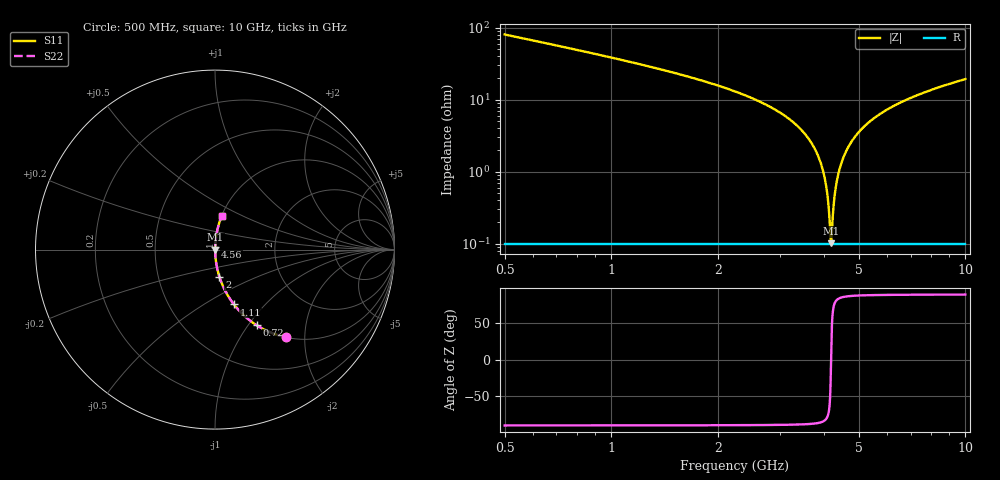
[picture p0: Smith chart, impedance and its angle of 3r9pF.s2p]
! Created Fri Jan 10 15:54:33 2014
# hz S db R 50
! 2 Port Network Data from SP1.SP block
! freq  dbS11  angS11  dbS21  angS21  dbS12  angS12  dbS22  angS22
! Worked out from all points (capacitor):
!   951 points, 500 MHz to 10 GHz, reference 50 ohm
!   read as one part in series: C = 3.9 pF near 540 MHz
!   lowest |Z| = 101 mohm at 4.18 GHz (marker M1)
!   series resonance near 4.176 GHz, so ESL is about 370 pH
!   S11 on the Smith chart (normalised r, x): 500 MHz: 1.00, -1.61; 720 MHz: 1.00, -1.10; 1.11 GHz: 1.00, -0.68; 2 GHz: 1.00, -0.31; 4.56 GHz: 1.00, +0.03; 10 GHz: 1.00, +0.39
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5e8  -4.06 -51.1  -2.17 38.8  -2.17 38.8  -4.06 -51.1
7.2e8  -6.35 -61.1  -1.15 28.8  -1.15 28.8  -6.35 -61.1
1.11e9  -9.82 -71.0  -0.49 18.8  -0.49 18.8  -9.82 -71.0
2e9  -16.18 -80.7  -0.11 8.9  -0.11 8.9  -16.18 -80.7
2.09e9  -16.79 -81.3  -0.10 8.3  -0.10 8.3  -16.79 -81.3
3.09e9  -24.50 -85.6  -0.02 3.4  -0.02 3.4  -24.50 -85.6
3.67e9  -31.94 -86.3  -0.01 1.4  -0.01 1.4  -31.94 -86.3
3.86e9  -36.25 -85.4  -0.01 0.9  -0.01 0.9  -36.25 -85.4
3.99e9  -40.97 -83.1  -0.01 0.5  -0.01 0.5  -40.97 -83.1
4.07e9  -45.85 -78.5  -0.01 0.3  -0.01 0.3  -45.85 -78.5
4.15e9  -56.15 -50.5  -0.01 0.1  -0.01 0.1  -56.15 -50.5
4.18e9  -59.92 11.6  -0.01 -0.0  -0.01 -0.0  -59.92 11.6
4.21e9  -54.51 58.2  -0.01 -0.1  -0.01 -0.1  -54.51 58.2
4.27e9  -46.99 77.0  -0.01 -0.2  -0.01 -0.2  -46.99 77.0
4.33e9  -42.90 81.7  -0.01 -0.4  -0.01 -0.4  -42.90 81.7
4.43e9  -38.72 84.4  -0.01 -0.7  -0.01 -0.7  -38.72 84.4
4.56e9  -35.27 85.7  -0.01 -1.0  -0.01 -1.0  -35.27 85.7
4.85e9  -30.65 86.4  -0.01 -1.7  -0.01 -1.7  -30.65 86.4
5.25e9  -26.92 86.2  -0.02 -2.6  -0.02 -2.6  -26.92 86.2
6.84e9  -20.01 83.7  -0.05 -5.7  -0.05 -5.7  -20.01 83.7
8.42e9  -16.66 81.2  -0.10 -8.4  -0.10 -8.4  -16.66 81.2
1e10  -14.45 78.8  -0.17 -10.9  -0.17 -10.9  -14.45 78.8
